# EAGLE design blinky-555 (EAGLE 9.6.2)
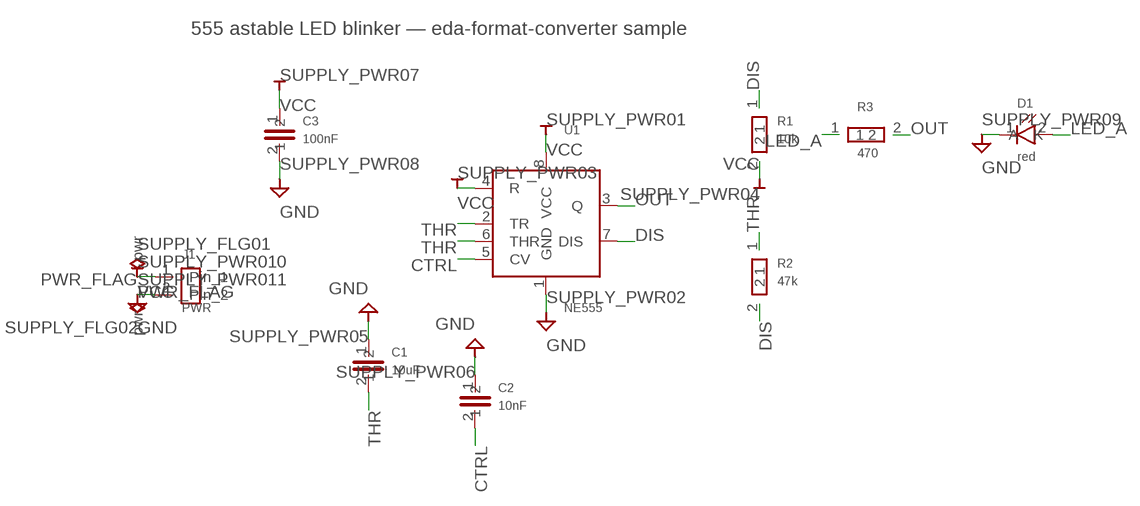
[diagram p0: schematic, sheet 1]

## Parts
C1  10uF  C  [C_PINS]
C2  10nF  C  [C_PINS]
C3  100nF  C  [C_PINS]
D1  red  LED  [LED_PINS]
J1  PWR  Conn_01x02  [PinHeader_1x02_P2.54mm_Vertical]
R1  10k  R  [R_PINS]
R2  47k  R  [R_PINS]
R3  470  R  [R_PINS]
SUPPLY_PWR01  VCC  (no package)
SUPPLY_PWR02  GND  (no package)
SUPPLY_PWR03  VCC  (no package)
SUPPLY_PWR04  VCC  (no package)
SUPPLY_PWR05  GND  (no package)
SUPPLY_PWR06  GND  (no package)
SUPPLY_PWR07  VCC  (no package)
SUPPLY_PWR08  GND  (no package)
SUPPLY_PWR09  GND  (no package)
SUPPLY_PWR010  VCC  (no package)
SUPPLY_PWR011  GND  (no package)
U1  NE555  [SOIC-8_3.9x4.9mm_P1.27mm]

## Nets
CTRL: C2.2 U1.5(CV)
DIS: R1.1 R2.2 U1.7(DIS)
GND: C1.1 C2.1 C3.2 D1.1(K) J1.2(Pin_2) SUPPLY_PWR02.GND SUPPLY_PWR05.GND SUPPLY_PWR06.GND SUPPLY_PWR08.GND SUPPLY_PWR09.GND SUPPLY_PWR011.GND U1.1(GND) ; supply symbol labelled PWR_FLAG
LED_A: D1.2(A) R3.1
OUT: R3.2 U1.3(Q)
THR: C1.2 R2.1 U1.2(TR) U1.6(THR)
VCC: C3.1 J1.1(Pin_1) R1.2 SUPPLY_PWR01.VCC SUPPLY_PWR03.VCC SUPPLY_PWR04.VCC SUPPLY_PWR07.VCC SUPPLY_PWR010.VCC U1.4(R) U1.8(VCC) ; supply symbol labelled PWR_FLAG

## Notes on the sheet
- 555 astable LED blinker — eda-format-converter sample

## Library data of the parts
C1-C3 = converted:C
D1 = converted:LED
J1 = converted:Conn_01x02
R1-R3 = converted:R
SUPPLY_PWR01 SUPPLY_PWR03 SUPPLY_PWR04 SUPPLY_PWR07 SUPPLY_PWR010 = converted:VCC
SUPPLY_PWR02 SUPPLY_PWR05 SUPPLY_PWR06 SUPPLY_PWR08 SUPPLY_PWR09 SUPPLY_PWR011 = converted:GND
U1 = converted:NE555: Precision timer

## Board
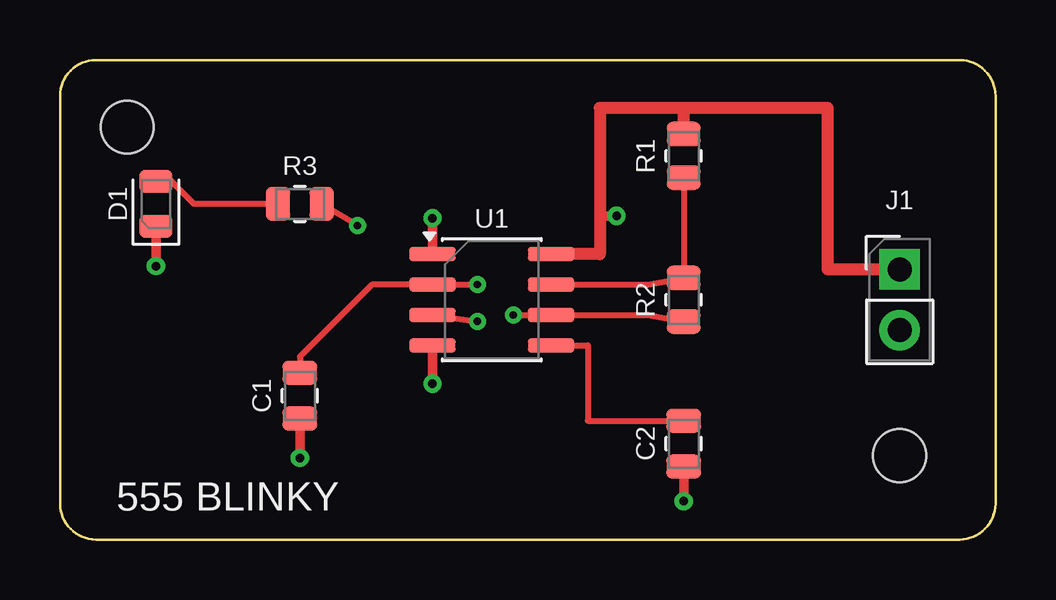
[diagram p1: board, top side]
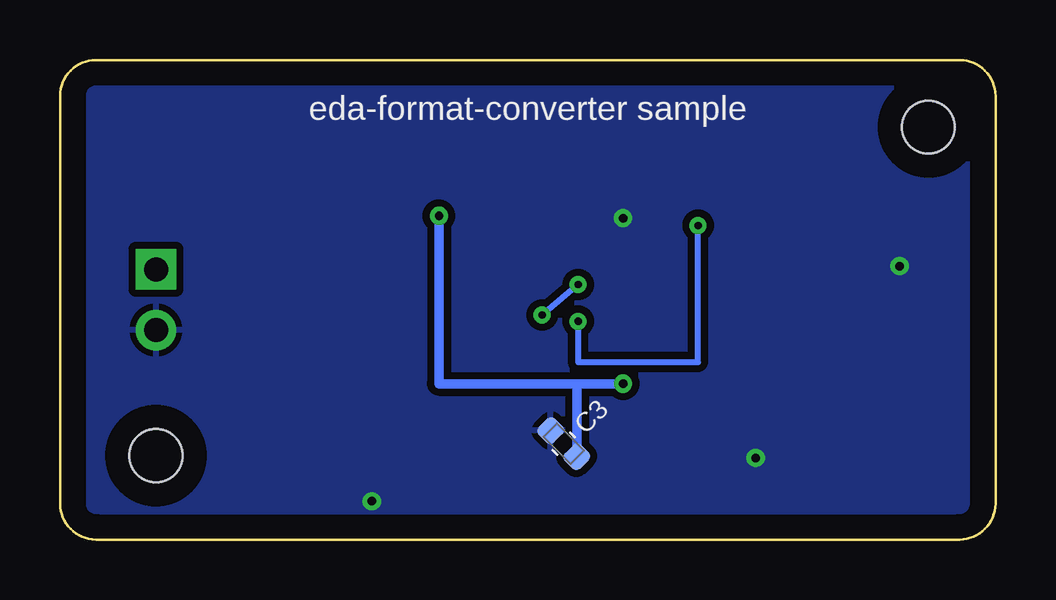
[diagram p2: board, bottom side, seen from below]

Size 39 x 20 mm. Coordinates in mm from the lower left corner, seen from the top.
Outline: 1.5,20 37.5,20 arc-90 39,18.5 39,1.5 arc-90 37.5,0 1.5,0 arc-90 0,1.5 0,18.5 arc-90 1.5,20
Copper layers (1*16): Top / Bottom
Holes 2.2 mm at 2.8,17.2 35,3.5

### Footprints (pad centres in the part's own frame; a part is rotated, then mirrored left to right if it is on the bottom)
C_0805_2012Metric = smd 1 x 1.45: 1 -0.95,0; 2 0.95,0
C_0603_1608Metric = smd 0.9 x 0.95: 1 0.775,0; 2 -0.775,0
LED_0805_2012Metric = smd 0.975 x 1.4: 1 -0.938,0; 2 0.938,0
PinHeader_1x02_P2.54mm_Vertical = drill 1 pad 1.7 square: 1 0,0 | drill 1 pad 1.7: 2 0,-2.54
R_0805_2012Metric = smd 1.025 x 1.4: 1 -0.912,0; 2 0.912,0
SOIC-8_3.9x4.9mm_P1.27mm = smd 1.95 x 0.6: 1 -2.475,1.905; 2 -2.475,0.635; 3 -2.475,-0.635; 4 -2.475,-1.905; 5 2.475,-1.905; 6 2.475,-0.635; 7 2.475,0.635; 8 2.475,1.905

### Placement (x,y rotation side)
C1  10uF  [C_0805_2012Metric]  10,6 90 top
C2  10nF  [C_0805_2012Metric]  26,4 90 top
C3  100nF  [C_0603_1608Metric]  18,4 315 bottom
D1  red  [LED_0805_2012Metric]  4,14 90 top
J1  35,11.27 0 top
R1  10k  [R_0805_2012Metric]  26,16 90 top
R2  47k  [R_0805_2012Metric]  26,10 90 top
R3  470  [R_0805_2012Metric]  10,14 0 top
U1  18,10 0 top

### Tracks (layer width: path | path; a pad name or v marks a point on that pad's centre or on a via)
CTRL
  Top 0.25: U1.5 22,8.09 22,4.95 C2.2
DIS
  Top 0.25: U1.7 24.5,10.63 R2.2 R1.1
GND  (via drill 0.35 pad 0.7)
  Top 0.4: U1.1 v15.52,13.4 | C1.1 v10,3.4 | C2.1 v26,1.6 | D1.1 v4,11.4
  pour Bottom (isolate 0.3): 0.5,19.5 38.5,19.5 38.5,0.5 0.5,0.5
LED_A
  Top 0.25: R3.1 5.6,14 4.66,14.94 D1.2
OUT  (via drill 0.3 pad 0.6)
  Top 0.25: U1.3 v17.4,9.1 | v12.4,13.1 R3.2
  Bottom 0.25: v17.4,9.1 17.4,7.4 12.4,7.4 v12.4,13.1
THR  (via drill 0.3 pad 0.6)
  Top 0.25: R2.1 24.5,9.36 U1.6 v18.9,9.36 | v17.4,10.63 U1.2 13,10.63 10,7.64 C1.2
  Bottom 0.25: v17.4,10.63 v18.9,9.36
VCC  (via drill 0.35 pad 0.7)
  Top 0.4: 22.5,13.5 v23.2,13.5 | U1.4 v15.52,6.5
  Top 0.5: J1.1 32,11.27 32,18 22.5,18 22.5,11.9 U1.8 | R1.2 26,18
  Bottom 0.4: v23.2,13.5 23.2,6.5 v15.52,6.5 | 17.45,6.5 C3.1

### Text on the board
tPlace: 555 BLINKY
bPlace: eda-format-converter sample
